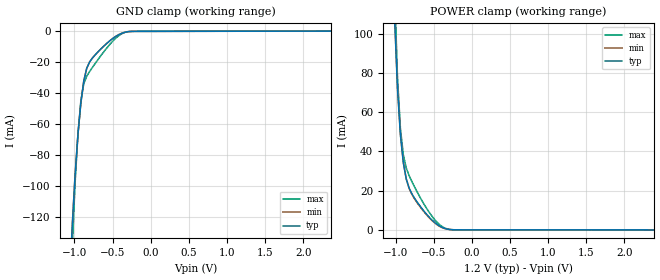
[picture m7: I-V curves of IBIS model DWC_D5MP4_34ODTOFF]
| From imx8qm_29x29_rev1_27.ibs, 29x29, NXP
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[Model] DWC_D5MP4_34ODTOFF
Model_type   Input
Polarity   Non-Inverting
Enable   Active-High
C_comp   1.264pF   1.181pF   1.264pF
C_comp_power_clamp   284.419fF   263.792fF   286.390fF
C_comp_gnd_clamp 969.046fF   901.845fF   969.654fF
Vinh = 910.000mV
Vinl = 724.000mV
[Model Spec]
D_overshoot_ampl_h 0.4 NA   NA
D_overshoot_ampl_l 0.4 NA   NA
D_overshoot_area_l 60.000p NA   NA
D_overshoot_area_h 60.000p NA   NA
[Receiver Thresholds]
Vth = 817.000mV
Vth_min = 805.000mV
Vth_max = 829.000mV
Vinh_ac = 68.000mV
Vinh_dc = 68.000mV
Vinl_ac = -68.000mV
Vinl_dc = -68.000mV
Tslew_ac = 5.000ns
Reference_supply Power_clamp_ref
[Temperature Range]   25.000   125.000   -40.000
[Voltage Range]   1.200V   1.140V   1.260V
[GND Clamp Reference]   0.00V   0.00V   0.00V
[C Comp Corner]
| variable   typ   min   max
C_comp 1.264pF   1.264pF   1.181pF
C_comp_pullup 284.419fF   286.390fF   263.792fF
C_comp_pulldown 969.046fF   969.654fF   901.845fF
[POWER Clamp Reference]   1.200V   1.140V   1.260V
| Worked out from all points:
|   GND clamp passes 1 mA (typ) near -0.36 V on its own axis
|   POWER clamp passes 1 mA (typ) near -0.38 V on its own axis
[GND Clamp]
-1.184V   -342.5mA   -342.4mA   -430.7mA
-1.031V   -127.6mA   -127.6mA   -142.7mA
-992.7mV  -93.59mA   -93.52mA   -98.99mA
-954.5mV  -66.78mA   -66.74mA   -66.61mA
-916.4mV  -46.35mA   -46.32mA   -45.02mA
-878.2mV  -32.2mA    -32.19mA   -34mA
-840mV    -24.05mA   -24.05mA   -29.18mA
-763.6mV  -17.22mA   -17.22mA   -23.29mA
-496.4mV  -4.559mA   -4.559mA   -6.292mA
-381.8mV  -1.286mA   -1.286mA   -1.614mA
-267.3mV  -89.24uA   -89.23uA   -59.9uA
2.367V    136.8uA    136.8uA    170.5uA
[Power Clamp]
-1.167V   370mA      370mA      475mA
-1.015V   108.4mA    109.7mA    123mA
-976.4mV  71.8mA     73.01mA    77.9mA
-938.2mV  48.37mA    49.08mA    51.81mA
-900mV    34.2mA     34.51mA    38.28mA
-861.8mV  25.98mA    25.98mA    31.54mA
-823.6mV  21.25mA    21.04mA    27.58mA
-747.3mV  15.81mA    15.45mA    21.46mA
-480mV    3.453mA    3.248mA    4.784mA
-365.5mV  823.4uA    745.6uA    1.073mA
-250.9mV  45.63uA    42.16uA    40.3uA
2.384V    -68.4uA    -71.86uA   -80.92uA
